FUNCTION_BLOCK "FB_CABINET_7P7-R23"
TITLE =Control cabinet 7P7-R23
{ S7_language := '9(1) Angielski (Stany Zjednoczone)  11.01.2022  09:45:15' }
VERSION : 0.1


VAR
  SM : STRUCT
   GeneralError : BOOL ;
   GeneralWarning : BOOL ;
   CtrlVoltageON : BOOL ;
   Auto : BOOL ;
   Manual : BOOL ;
   Local : BOOL ;
   Remote : BOOL ;
   CtrlRelease : BOOL ;
   CtrlRelease_A : BOOL ;
   res11 : BOOL ;
   res12 : BOOL ;
   res13 : BOOL ;
   res14 : BOOL ;
   res15 : BOOL ;
   LackCooling : BOOL ;
   LackHeating : BOOL ;
  END_STRUCT ;
  FM : STRUCT
   EnergyCounterFuse : BOOL ;
   ControlVoltage230VAC : BOOL ;
   ControlVoltage24VDC : BOOL ;
   ControlVoltage230VAC_MS : BOOL ;
   CabinetCoolingFuse : BOOL ;
   ProfiNetSwitchFault : BOOL ;
   MainSwitchFault : BOOL ;
   ExcessTemperature : BOOL ;
   ESTOP : BOOL ;
   FireAlarmPreWarning : BOOL ;
   FireAlarm : BOOL ;
   res13 : BOOL ;
   res14 : BOOL ;
   res15 : BOOL ;
   res16 : BOOL ;
   res17 : BOOL ;
  END_STRUCT ;
  CTRL : STRUCT
   ResetFault : BOOL ;
   ResetESTOP : BOOL ;
   LampTest : BOOL ;
   AutoStart : BOOL ;
   AutoStop : BOOL ;
   res05 : BOOL ;
   res06 : BOOL ;
   res07 : BOOL ;
   res10 : BOOL ;
   res11 : BOOL ;
   res12 : BOOL ;
   res13 : BOOL ;
   res14 : BOOL ;
   res15 : BOOL ;
   res16 : BOOL ;
   res17 : BOOL ;
  END_STRUCT ;
  CTRL_HMI : STRUCT
   ResetFault : BOOL ;
   Auto : BOOL ;
   Manual : BOOL ;
   res03 : BOOL ;
   res04 : BOOL ;
   res05 : BOOL ;
   res06 : BOOL ;
   res07 : BOOL ;
   ProductionOn : BOOL ;
   ProductionBreak : BOOL ;
   PlantOn : BOOL ;
   PlantOff : BOOL ;
   res14 : BOOL ;
   res15 : BOOL ;
   LackCooling : BOOL ;
   LackHeating : BOOL ;
  END_STRUCT ;
  EC : "UDT_EC";	//Energy Counter
END_VAR
VAR_TEMP
  ERROR_REL : BOOL ;
END_VAR
BEGIN
NETWORK
TITLE =STATUS



NETWORK
TITLE =CONTROL VOLTAGE ON
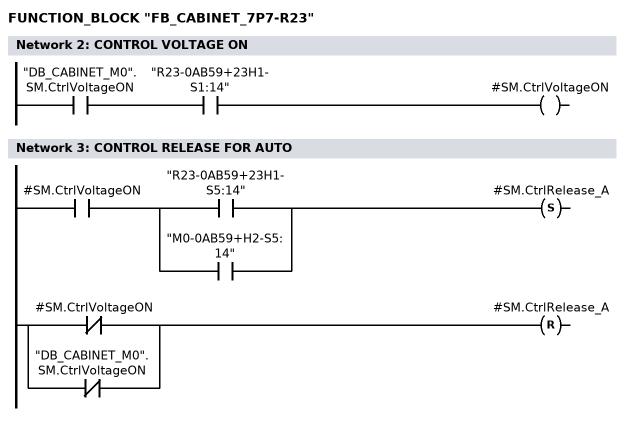
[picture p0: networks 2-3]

      U     "DB_CABINET_M0".SM.CtrlVoltageON;
      U     "R23-0AB59+23H1-S1:14";
      =     #SM.CtrlVoltageON;
NETWORK
TITLE =CONTROL RELEASE FOR AUTO

      U     #SM.CtrlVoltageON;
      U(    ;
      O     "R23-0AB59+23H1-S5:14";
      O     "M0-0AB59+H2-S5:14";
      )     ;
      S     #SM.CtrlRelease_A;
      U(    ;
      ON    #SM.CtrlVoltageON;
      ON    "DB_CABINET_M0".SM.CtrlVoltageON;
      )     ;
      R     #SM.CtrlRelease_A;
      NOP   0;
NETWORK
TITLE =AUTO/MANUAL MODE

      U(    ;
      U     "R23-0AB59+23H1-S2:14";
      S     #SM.Auto;
      U     "R23-0AB59+23H1-S2:22";
      R     #SM.Auto;
      U     #SM.Auto;
      )     ;
      NOT   ;
      =     #SM.Manual;
NETWORK
TITLE =LOCAL/REMOTE MODE

      U(    ;
      U     "DB_CABINET_M0".SM.Remote;
      S     #SM.Remote;
      U     "DB_CABINET_M0".SM.Local;
      R     #SM.Remote;
      U     #SM.Remote;
      )     ;
      NOT   ;
      =     #SM.Local;
NETWORK
TITLE =CONTROL RELEASE FROM CABINET
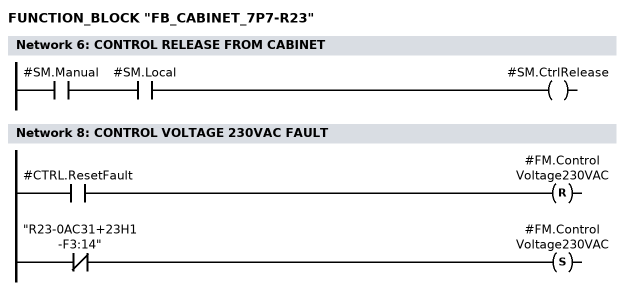
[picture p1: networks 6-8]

      U     #SM.Manual;
      U     #SM.Local;
      =     #SM.CtrlRelease;
NETWORK
TITLE =FAULTS



NETWORK
TITLE =CONTROL VOLTAGE 230VAC FAULT

      U     #CTRL.ResetFault;
      R     #FM.ControlVoltage230VAC;
      UN    "R23-0AC31+23H1-F3:14";
      S     #FM.ControlVoltage230VAC;
      NOP   0;
NETWORK
TITLE =CONTROL VOLTAGE 24V DC FAULT

      U     #CTRL.ResetFault;
      R     #FM.ControlVoltage24VDC;
      U(    ;
      O(    ;
      UN    "R23-0DC43+23H2-F1:7";
      L     S5T#300MS;
      SE    "T_R23-0DC43+23H2-F1";
      NOP   0;
      NOP   0;
      NOP   0;
      U     "T_R23-0DC43+23H2-F1";
      )     ;
      O(    ;
      UN    "R23-0DC43+23H2-F2:7";
      L     S5T#300MS;
      SE    "T_R23-0DC43+23H2-F2";
      NOP   0;
      NOP   0;
      NOP   0;
      U     "T_R23-0DC43+23H2-F2";
      )     ;
      )     ;
      S     #FM.ControlVoltage24VDC;
      NOP   0;
NETWORK
TITLE =CONTROL VOLTAGE 230V AC BEFORE MAIN SWITCH FAULT
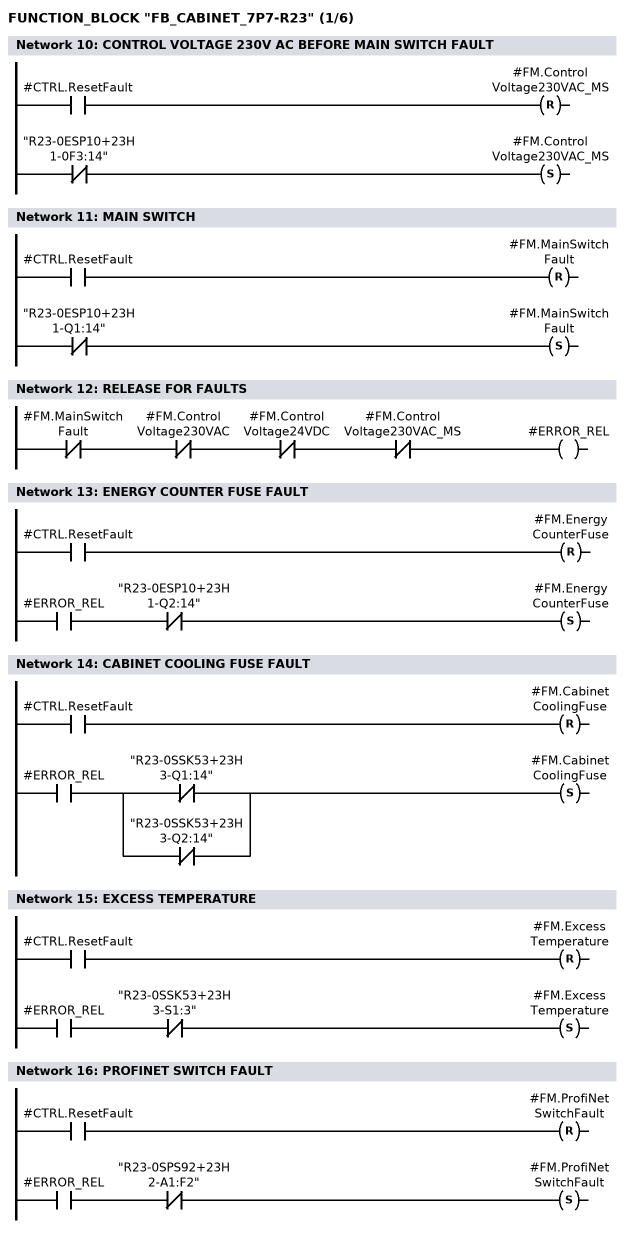
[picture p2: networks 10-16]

      U     #CTRL.ResetFault;
      R     #FM.ControlVoltage230VAC_MS;
      UN    "R23-0ESP10+23H1-0F3:14";
      S     #FM.ControlVoltage230VAC_MS;
      NOP   0;
NETWORK
TITLE =MAIN SWITCH

      U     #CTRL.ResetFault;
      R     #FM.MainSwitchFault;
      UN    "R23-0ESP10+23H1-Q1:14";
      S     #FM.MainSwitchFault;
      NOP   0;
NETWORK
TITLE =RELEASE FOR FAULTS

      UN    #FM.MainSwitchFault;
      UN    #FM.ControlVoltage230VAC;
      UN    #FM.ControlVoltage24VDC;
      UN    #FM.ControlVoltage230VAC_MS;
      =     #ERROR_REL;
NETWORK
TITLE =ENERGY COUNTER FUSE FAULT

      U     #CTRL.ResetFault;
      R     #FM.EnergyCounterFuse;
      U     #ERROR_REL;
      UN    "R23-0ESP10+23H1-Q2:14";
      S     #FM.EnergyCounterFuse;
      NOP   0;
NETWORK
TITLE =CABINET COOLING FUSE FAULT

      U     #CTRL.ResetFault;
      R     #FM.CabinetCoolingFuse;
      U     #ERROR_REL;
      U(    ;
      ON    "R23-0SSK53+23H3-Q1:14";
      ON    "R23-0SSK53+23H3-Q2:14";
      )     ;
      S     #FM.CabinetCoolingFuse;
      NOP   0;
NETWORK
TITLE =EXCESS TEMPERATURE

      U     #CTRL.ResetFault;
      R     #FM.ExcessTemperature;
      U     #ERROR_REL;
      UN    "R23-0SSK53+23H3-S1:3";
      S     #FM.ExcessTemperature;
      NOP   0;
NETWORK
TITLE =PROFINET SWITCH FAULT

      U     #CTRL.ResetFault;
      R     #FM.ProfiNetSwitchFault;
      U     #ERROR_REL;
      UN    "R23-0SPS92+23H2-A1:F2";
      S     #FM.ProfiNetSwitchFault;
      NOP   0;
NETWORK
TITLE =ESTOP FAULT
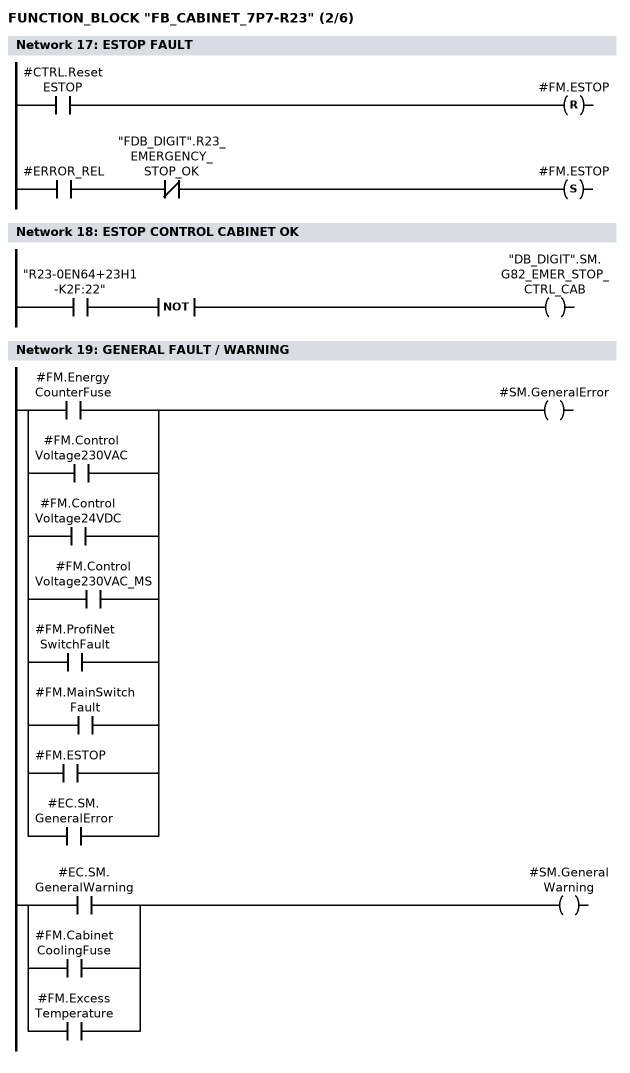
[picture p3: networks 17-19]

      U     #CTRL.ResetESTOP;
      R     #FM.ESTOP;
      U     #ERROR_REL;
      UN    "FDB_DIGIT".R23_EMERGENCY_STOP_OK;
      S     #FM.ESTOP;
      NOP   0;
NETWORK
TITLE =ESTOP CONTROL CABINET OK

      U     "R23-0EN64+23H1-K2F:22";
      NOT   ;
      =     "DB_DIGIT".SM.G82_EMER_STOP_CTRL_CAB;
NETWORK
TITLE =GENERAL FAULT / WARNING


      U     #FM.EnergyCounterFuse;
      O     #FM.ControlVoltage230VAC;
      O     #FM.ControlVoltage24VDC;
      O     #FM.ControlVoltage230VAC_MS;
      O     #FM.ProfiNetSwitchFault;
      O     #FM.MainSwitchFault;
      O     #FM.ESTOP;
      O     #EC.SM.GeneralError;
      =     #SM.GeneralError;


      U     #EC.SM.GeneralWarning;
      O     #FM.CabinetCoolingFuse;
      O     #FM.ExcessTemperature;
      =     #SM.GeneralWarning;

NETWORK
TITLE =CONTROL SIGNALS



NETWORK
TITLE =RESET FAULT
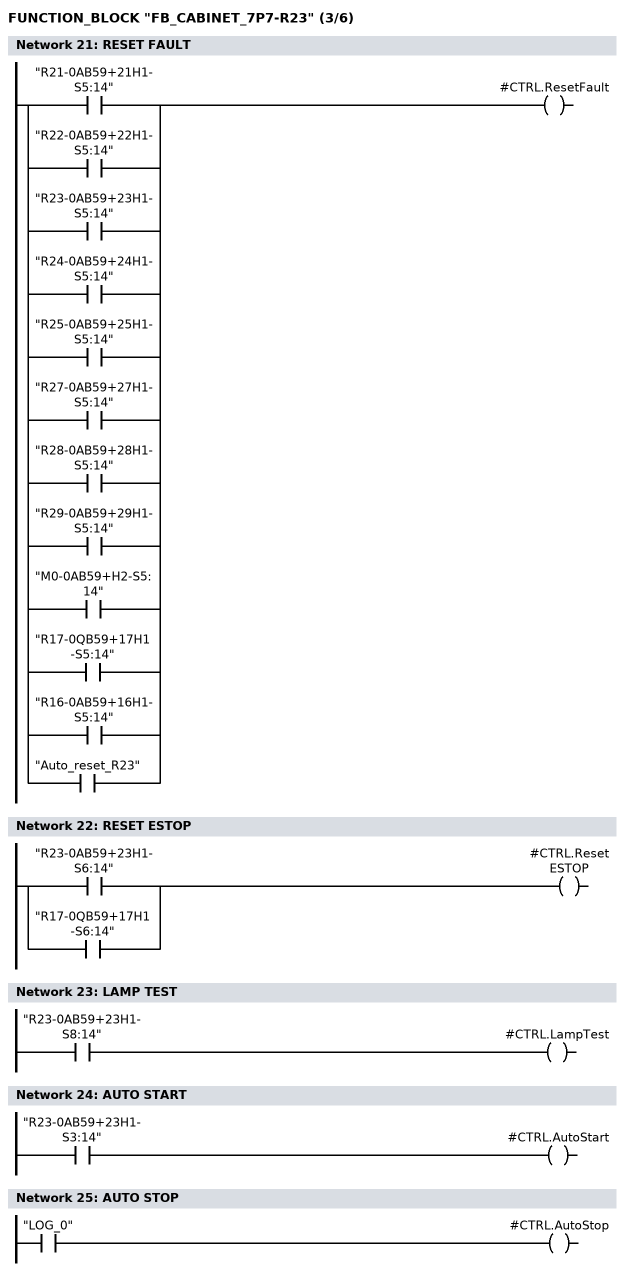
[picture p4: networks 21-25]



      O     "R21-0AB59+21H1-S5:14";
      O     "R22-0AB59+22H1-S5:14";
      O     "R23-0AB59+23H1-S5:14";
      O     "R24-0AB59+24H1-S5:14";
      O     "R25-0AB59+25H1-S5:14";
      O     "R27-0AB59+27H1-S5:14";
      O     "R28-0AB59+28H1-S5:14";
      O     "R29-0AB59+29H1-S5:14";
      O     "M0-0AB59+H2-S5:14";
      O     "R17-0QB59+17H1-S5:14";
      O     "R16-0AB59+16H1-S5:14";
      O     "Auto_reset_R23";
      =     #CTRL.ResetFault;
NETWORK
TITLE =RESET ESTOP



      O     "R23-0AB59+23H1-S6:14";
      O     "R17-0QB59+17H1-S6:14";
      =     #CTRL.ResetESTOP;
NETWORK
TITLE =LAMP TEST



      U     "R23-0AB59+23H1-S8:14";
      =     #CTRL.LampTest;
NETWORK
TITLE =AUTO START



      U     "R23-0AB59+23H1-S3:14";
      =     #CTRL.AutoStart;
NETWORK
TITLE =AUTO STOP



      U     "LOG_0";
      =     #CTRL.AutoStop;
NETWORK
TITLE =BUTTON LAMPS
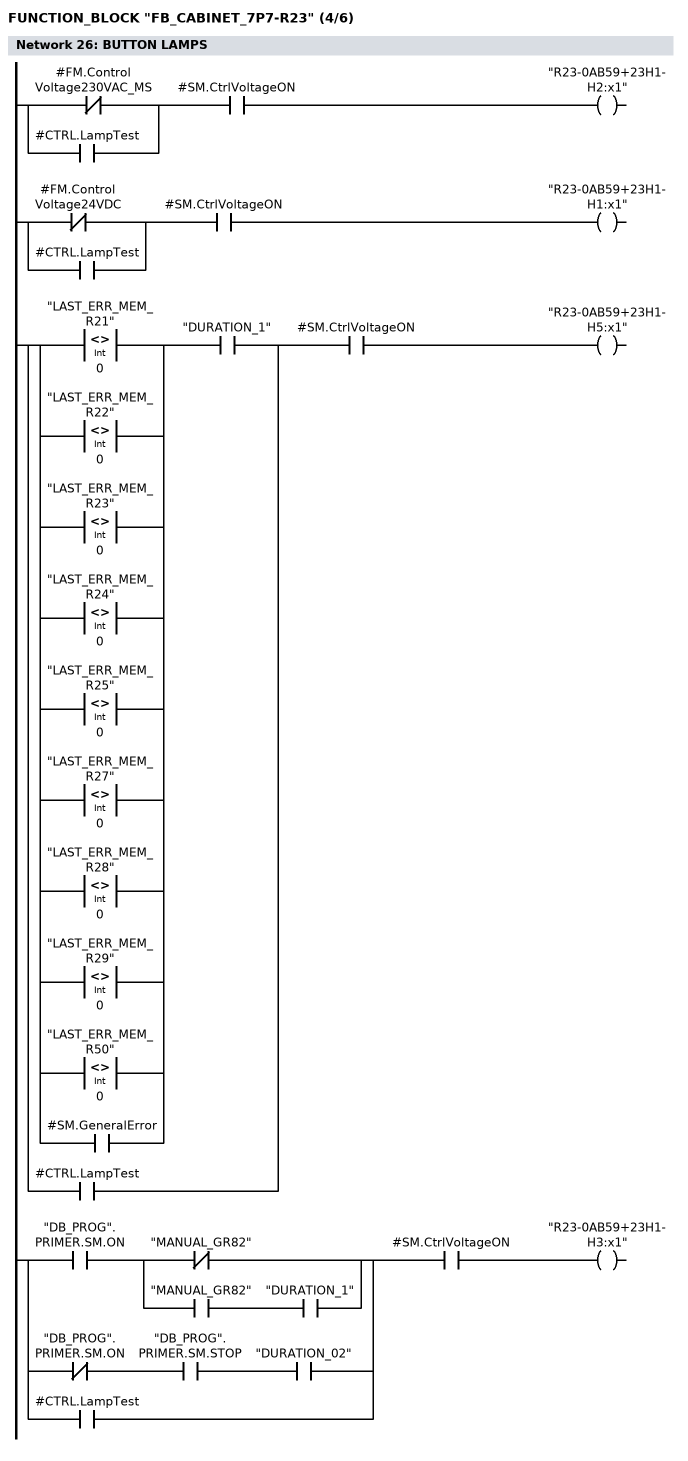
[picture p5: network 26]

// CONTROL VOLTAGE 230V AC
      U(    ;
      ON    #FM.ControlVoltage230VAC_MS;
      O     #CTRL.LampTest;
      )     ;
      U     #SM.CtrlVoltageON;
      =     "R23-0AB59+23H1-H2:x1";

// CONTROL VOLTAGE 24V DC
      U(    ;
      ON    #FM.ControlVoltage24VDC;
      O     #CTRL.LampTest;
      )     ;
      U     #SM.CtrlVoltageON;
      =     "R23-0AB59+23H1-H1:x1";

// RESET
      U(    ;
      L     "LAST_ERR_MEM_R21";
      L     0;
      <>I   ;
      )     ;
      O(    ;
      L     "LAST_ERR_MEM_R22";
      L     0;
      <>I   ;
      )     ;
      O(    ;
      L     "LAST_ERR_MEM_R23";
      L     0;
      <>I   ;
      )     ;
      O(    ;
      L     "LAST_ERR_MEM_R24";
      L     0;
      <>I   ;
      )     ;
      O(    ;
      L     "LAST_ERR_MEM_R25";
      L     0;
      <>I   ;
      )     ;
      O(    ;
      L     "LAST_ERR_MEM_R27";
      L     0;
      <>I   ;
      )     ;
      O(    ;
      L     "LAST_ERR_MEM_R28";
      L     0;
      <>I   ;
      )     ;
      O(    ;
      L     "LAST_ERR_MEM_R29";
      L     0;
      <>I   ;
      )     ;
      O(    ;
      L     "LAST_ERR_MEM_R50";
      L     0;
      <>I   ;
      )     ;
      O     #SM.GeneralError;
      U     "DURATION_1";
      O     #CTRL.LampTest;
      U     #SM.CtrlVoltageON;
      =     "R23-0AB59+23H1-H5:x1";

// AUTOMATIC START
      U(    ;
      U     "DB_PROG".PRIMER.SM.ON;
      U(    ;
      ON    "MANUAL_GR82";
      O     ;
      U     "MANUAL_GR82";
      U     "DURATION_1";
      )     ;
      O     ;
      UN    "DB_PROG".PRIMER.SM.ON;
      U     "DB_PROG".PRIMER.SM.STOP;
      U     "DURATION_02";
      O     #CTRL.LampTest;
      )     ;
      U     #SM.CtrlVoltageON;

      =     "R23-0AB59+23H1-H3:x1";
NETWORK
TITLE =LIGHT TOWER
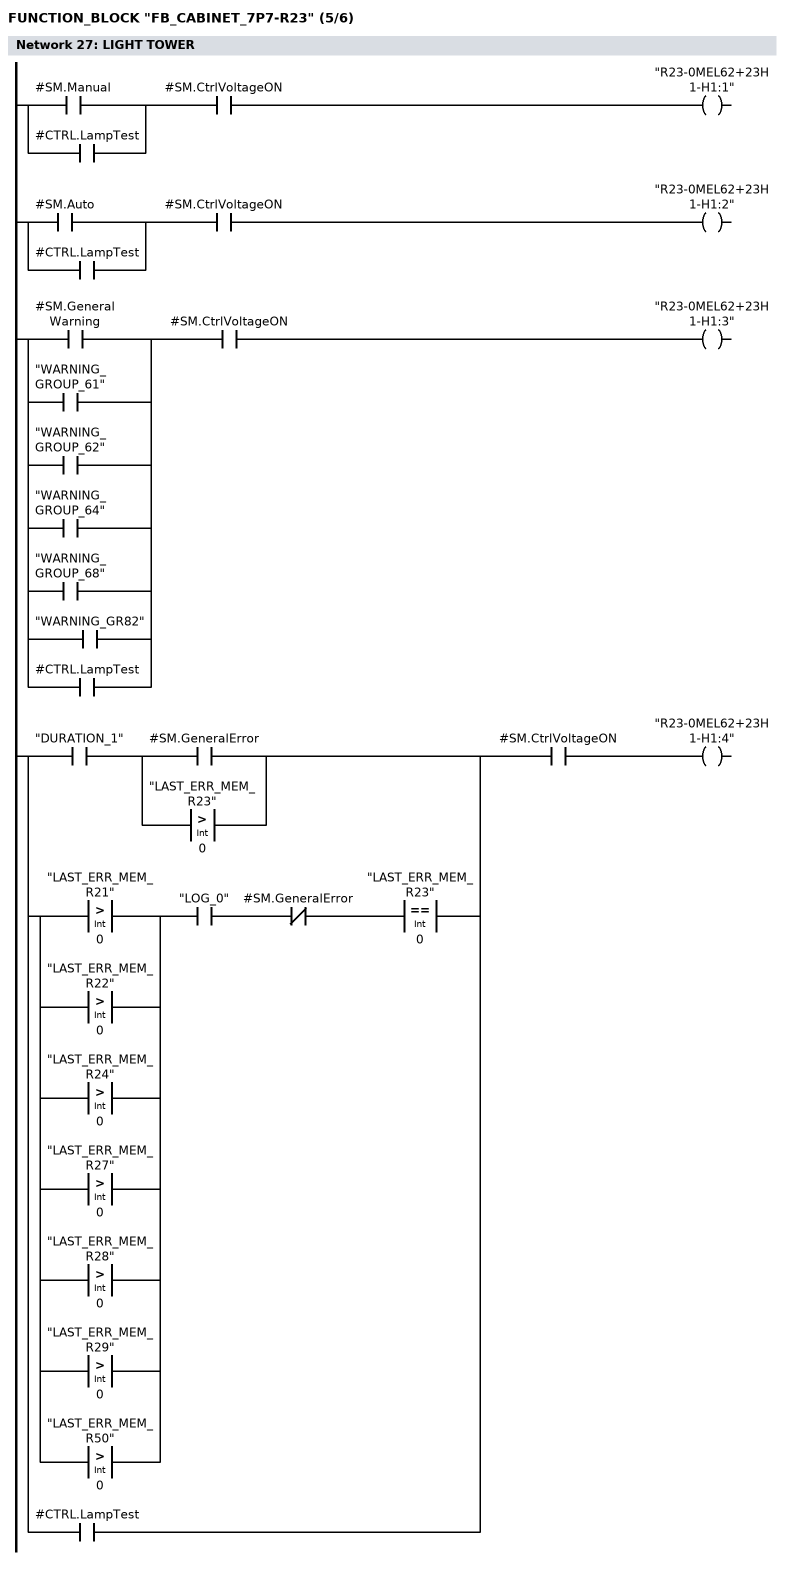
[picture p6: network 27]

// MANUAL
      U(    ;
      O     #SM.Manual;
      O     #CTRL.LampTest;
      )     ;
      U     #SM.CtrlVoltageON;
      =     "R23-0MEL62+23H1-H1:1";

// AUTO
      U(    ;
      O     #SM.Auto;
      O     #CTRL.LampTest;
      )     ;
      U     #SM.CtrlVoltageON;
      =     "R23-0MEL62+23H1-H1:2";

// WARNING
      U(    ;
      O     #SM.GeneralWarning;
      O     "WARNING_GROUP_61";
      O     "WARNING_GROUP_62";
      O     "WARNING_GROUP_64";
      O     "WARNING_GROUP_68";
      O     "WARNING_GR82";
      O     #CTRL.LampTest;
      )     ;
      U     #SM.CtrlVoltageON;
      =     "R23-0MEL62+23H1-H1:3";

// FAULT
      U(    ;
      U     "DURATION_1";
      U(    ;
      O     #SM.GeneralError;
      O(    ;
      L     "LAST_ERR_MEM_R23";
      L     0;
      >I    ;
      )     ;
      )     ;
      O     ;
      U(    ;
      O(    ;
      L     "LAST_ERR_MEM_R21";
      L     0;
      >I    ;
      )     ;
      O(    ;
      L     "LAST_ERR_MEM_R22";
      L     0;
      >I    ;
      )     ;
      O(    ;
      L     "LAST_ERR_MEM_R24";
      L     0;
      >I    ;
      )     ;
      O(    ;
      L     "LAST_ERR_MEM_R27";
      L     0;
      >I    ;
      )     ;
      O(    ;
      L     "LAST_ERR_MEM_R28";
      L     0;
      >I    ;
      )     ;
      O(    ;
      L     "LAST_ERR_MEM_R29";
      L     0;
      >I    ;
      )     ;
      O(    ;
      L     "LAST_ERR_MEM_R50";
      L     0;
      >I    ;
      )     ;
      )     ;
      U     "LOG_0";
      UN    #SM.GeneralError;
      U(    ;
      L     "LAST_ERR_MEM_R23";
      L     0;
      ==I   ;
      )     ;
      O     #CTRL.LampTest;
      )     ;
      U     #SM.CtrlVoltageON;

      =     "R23-0MEL62+23H1-H1:4";
NETWORK
TITLE =HORN
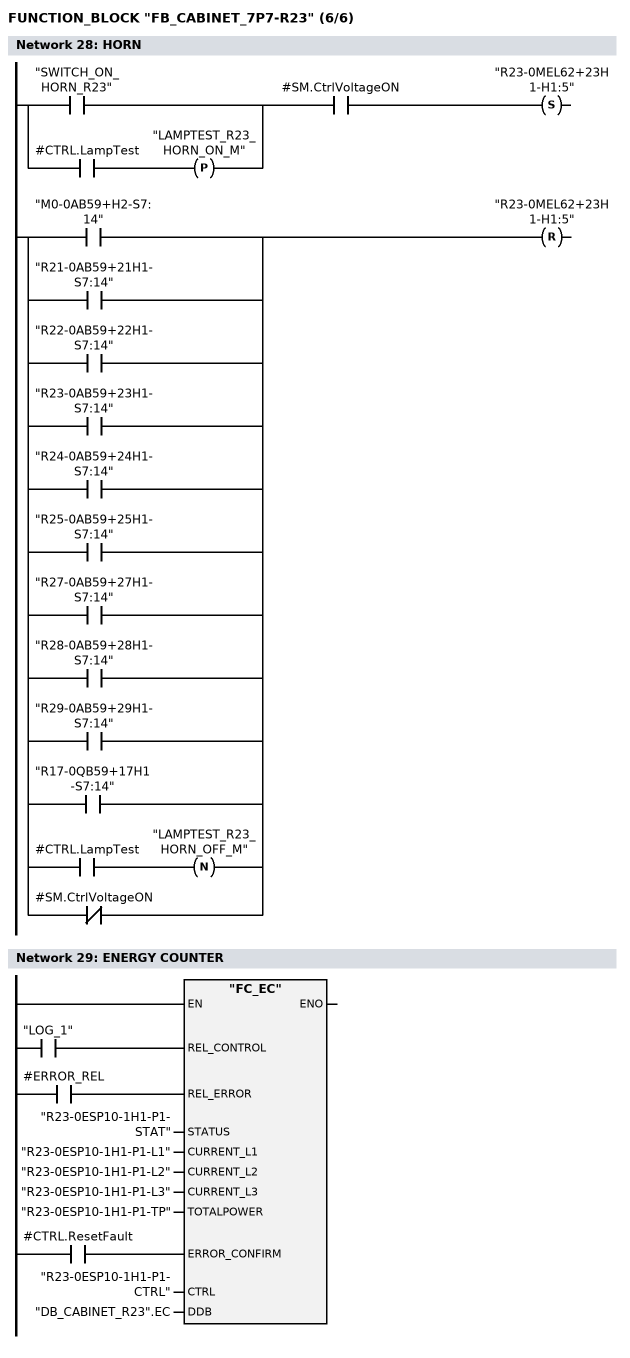
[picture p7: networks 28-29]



      U(    ;
      O     "SWITCH_ON_HORN_R23";
      O(    ;
      U     #CTRL.LampTest;
      FP    "LAMPTEST_R23_HORN_ON_M";
      )     ;
      )     ;
      U     #SM.CtrlVoltageON;
      S     "R23-0MEL62+23H1-H1:5";
      U(    ;
      O     "M0-0AB59+H2-S7:14";
      O     "R21-0AB59+21H1-S7:14";
      O     "R22-0AB59+22H1-S7:14";
      O     "R23-0AB59+23H1-S7:14";
      O     "R24-0AB59+24H1-S7:14";
      O     "R25-0AB59+25H1-S7:14";
      O     "R27-0AB59+27H1-S7:14";
      O     "R28-0AB59+28H1-S7:14";
      O     "R29-0AB59+29H1-S7:14";
      O     "R17-0QB59+17H1-S7:14";
      O(    ;
      U     #CTRL.LampTest;
      FN    "LAMPTEST_R23_HORN_OFF_M";
      )     ;
      ON    #SM.CtrlVoltageON;
      )     ;
      R     "R23-0MEL62+23H1-H1:5";
      NOP   0;
NETWORK
TITLE =ENERGY COUNTER

      U     "LOG_1";
      =     L      1.0;
      BLD   103;
      U     #ERROR_REL;
      =     L      1.1;
      BLD   103;
      U     #CTRL.ResetFault;
      =     L      1.2;
      BLD   103;
      CALL "FC_EC" (
           REL_CONTROL              := L      1.0,
           REL_ERROR                := L      1.1,
           STATUS                   := "R23-0ESP10-1H1-P1-STAT",
           CURRENT_L1               := "R23-0ESP10-1H1-P1-L1",
           CURRENT_L2               := "R23-0ESP10-1H1-P1-L2",
           CURRENT_L3               := "R23-0ESP10-1H1-P1-L3",
           TOTALPOWER               := "R23-0ESP10-1H1-P1-TP",
           ERROR_CONFIRM            := L      1.2,
           CTRL                     := "R23-0ESP10-1H1-P1-CTRL",
           DDB                      := "DB_CABINET_R23".EC);
      NOP   0;
NETWORK
TITLE =END

END_FUNCTION_BLOCK

